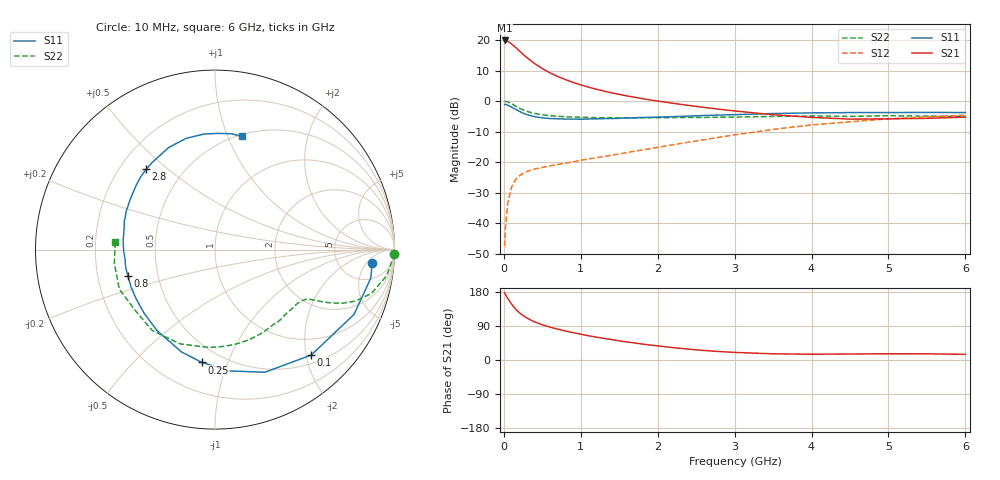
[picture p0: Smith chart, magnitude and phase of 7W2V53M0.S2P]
! Infineon Technologies  Discrete & RF Semiconductors
! BFS17W
! Si NPN RF Bipolar Junction Transistor in SOT323
! VCE = 2.5 V  IC = 3 mA
! Common Emitter S-Parameters:  August  1999
# GHz  S  MA  R  50
!  f  S11  S21  S12  S22
! GHz  MAG  ANG  MAG  ANG  MAG  ANG  MAG  ANG
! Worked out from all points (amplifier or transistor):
!   36 points, 10 MHz to 6 GHz, reference 50 ohm
!   highest |S21| = 19.8 dB at 10 MHz (marker M1)
!   |S21| within 3 dB of that: start of sweep to 184.3 MHz
!   unconditionally stable (mu >= 1): 690.5 MHz to end of sweep
!   at 250 MHz: K = 0.45, MSG = 19.5 dB, |S12| = -23.7 dB
!   at 1.4 GHz: K = 1.30, MAG = 6.9 dB, |S12| = -17.7 dB
!   at 6 GHz: K = 1.10, MAG = -2.2 dB, |S12| = -4.6 dB
!   S11 on the Smith chart (normalised r, x): 10 MHz: 11, -7; 100 MHz: 0.66, -2.10; 250 MHz: 0.39, -0.81; 800 MHz: 0.33, -0.13; 2.8 GHz: 0.31, +0.42; 6 GHz: 0.52, +1.12
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0.01  0.8792 -5.0  9.828 177.1  0.0042 82.7  0.997 -1.3
0.02  0.8822 -10.4  9.778 173.0  0.0083 81.0  0.9898 -3.5
0.05  0.8547 -25.0  9.513 162.6  0.0211 76.7  0.9679 -8.6
0.1  0.7954 -47.6  8.634 147.7  0.039 65.7  0.906 -15.6
0.15  0.7376 -67.9  7.632 134.7  0.0514 56.8  0.832 -20.2
0.2  0.6801 -83.5  6.669 125.0  0.0597 51.8  0.7687 -22.9
0.25  0.6326 -96.6  5.82 117.1  0.0655 47.1  0.7172 -24.5
0.3  0.6003 -108.0  5.136 110.7  0.0703 45.1  0.679 -25.6
0.4  0.5553 -125.5  4.107 100.5  0.0769 42.6  0.6258 -26.8
0.5  0.5305 -138.3  3.405 93.0  0.0819 42.4  0.5961 -27.7
0.6  0.5177 -148.3  2.893 86.7  0.087 43.3  0.5759 -28.8
0.8  0.5069 -163.2  2.247 76.5  0.0962 45.8  0.5529 -32.2
0.9  0.5075 -168.9  2.017 72.2  0.1011 47.2  0.5457 -34.0
1.1  0.5085 -178.9  1.69 64.0  0.1129 49.9  0.5389 -38.4
1.3  0.5155 172.6  1.459 57.0  0.1241 53.0  0.5323 -43.5
1.6  0.5301 162.5  1.213 47.6  0.1431 56.4  0.5301 -51.4
2.2  0.5551 145.9  0.919 32.7  0.1927 61.2  0.5366 -69.1
2.8  0.5892 130.6  0.734 22.3  0.2551 61.4  0.543 -87.9
3.5  0.6243 114.5  0.597 16.3  0.3435 57.5  0.5602 -110.3
4.5  0.6469 95.5  0.506 15.8  0.457 45.8  0.5595 -143.6
5.5  0.652 81.8  0.521 16.3  0.5508 33.5  0.5659 -172.1
6  0.6481 76.7  0.545 14.9  0.5879 27.6  0.5582 175.5
